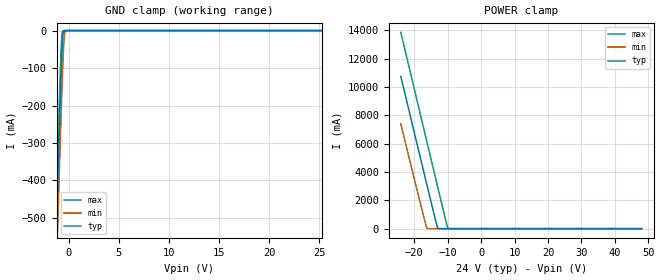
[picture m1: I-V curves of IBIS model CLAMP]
| Texas Instruments Incorporated
| 33V Precision Surge Protection Clamp
| Marketing part#   Voltage Range   Package-type   #pins/pkg drawing
| TVS3300YZF   21.6V - 26.4V   BGA   4 BGA YZF
[IBIS Ver]   4.1
[File name]   tvs3300.ibs
[File Rev]   1.0
[Date]   12/10/2016
[Source]   Model built from spectre simulations at:
   Texas Instruments Incorporated.
   Webench Design Center
   12500 TI Blvd
   Dallas, TX -75243
   For Support e-mail: elab_ibis@list.ti.com
[Notes]   Revision History
   Rev 1.0: 12/10/2016
   - ccomp values are based bench measuremets:
   Min and Max are 20% variation from nominal to account for PVT variations
[Disclaimer]  This model is designed as an aid for customers of Texas Instruments
 TI and its licensors and suppliers make no warranties, either expressed
 or implied, with respect to this  model, including the warranties of
 merchantability or fitness for a particular purpose.
 The model is provided solely on an "as is" basis. The entire risk as to
 its quality and performance is with the customer.
[Copyright] (C)Copyright 2016 Texas Instruments Incorporated.
   All rights reserved.
[Component]   TVS3300YZF
[Manufacturer]  Texas Instruments Incorporated
[Package]   |4-pin BGA YZF package
|   typ   min   max
R_pkg   0.005   0.005   0.005
L_pkg   0.20nH   0.2nH   0.2nH
C_pkg   0.6pF   0.6pF   0.6pF
[Pin]   signal_name   model_name   R_pin   L_pin   C_pin
A1   GND   GND   0.005   0.2nH   0.6pF
A2   GND   GND   0.005   0.2nH   0.6pF
A3   IN   CLAMP   0.005   0.2nH   0.6pF
A4   IN   CLAMP   0.005   0.2nH   0.6pF
[Component]   TVS3300DRV
[Manufacturer]  Texas Instruments Incorporated
[Package]   |6-pin SON DRV package
|   typ   min   max
R_pkg   0.03312   0.03141   0.03462
L_pkg   0.49614nH   0.44882nH   0.53669nH
C_pkg   0.15951pF   0.15201pF   0.17090pF
[Pin]   signal_name   model_name   R_pin   L_pin   C_pin
1   GND   GND   0.03462  0.53669n  0.15967p
2   GND   GND   0.03413  0.51329n  0.17090p
3   GND   GND   0.03462  0.53413n  0.15862p
4   IN   CLAMP   0.03197  0.47338n  0.15259p
5   IN   CLAMP   0.03141  0.44882n  0.16329p
6   IN   CLAMP   0.03197  0.47054n  0.15201p
| Models and submodels in the file (1): CLAMP (Terminator)
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|   Model CLAMP
[Model]   CLAMP
Model_type   Terminator
|   typ   min   max
C_comp   130p   104p   156p
[Voltage Range]   24   21.6   26.4
[Temperature Range]   27   125   -40
[Power Clamp Reference]   24   21.6   26.4
[GND Clamp Reference]   0   0   0
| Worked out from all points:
|   GND clamp passes 1 mA (typ) near -0.47 V on its own axis
|   POWER clamp passes 1 mA (typ) near -12.85 V on its own axis
[GND Clamp]
|   Voltage   I(typ)   I(min)   I(max)
-24V      -22.75A    -22.76A    -22.76A
-1.32V    -626.3mA   -734.6mA   -556.4mA
-1.248V   -560.4mA   -669mA     -490.1mA
-1.176V   -494.8mA   -603.6mA   -424.2mA
-1.032V   -365mA     -474.2mA   -294mA
-744mV    -118.6mA   -224.3mA   -53.06mA
-672mV    -65.06mA   -165.8mA   -12.89mA
-600mV    -22.7mA    -110.6mA   -1.204mA
-528mV    -3.22mA    -61.57mA   -152.7uA
-384mV    -116.1uA   -5.441mA   0A
-96mV     0A         0A         0A
48V       0A         0A         0A
[POWER Clamp]
|   Voltage   I(typ)   I(min)   I(max)
-24V      10.74A     7.393A     13.85A
-17.88V   4.731A     1.523A     7.784A
-16.22V   3.113A     52.37mA    6.146A
-15.94V   2.833A     354.7uA    5.861A
-12.98V   37.87mA    0A         2.948A
-10.54V   0A         0A         553.2mA
-9.888V   0A         0A         1.361mA
48V       0A         0A         0A
